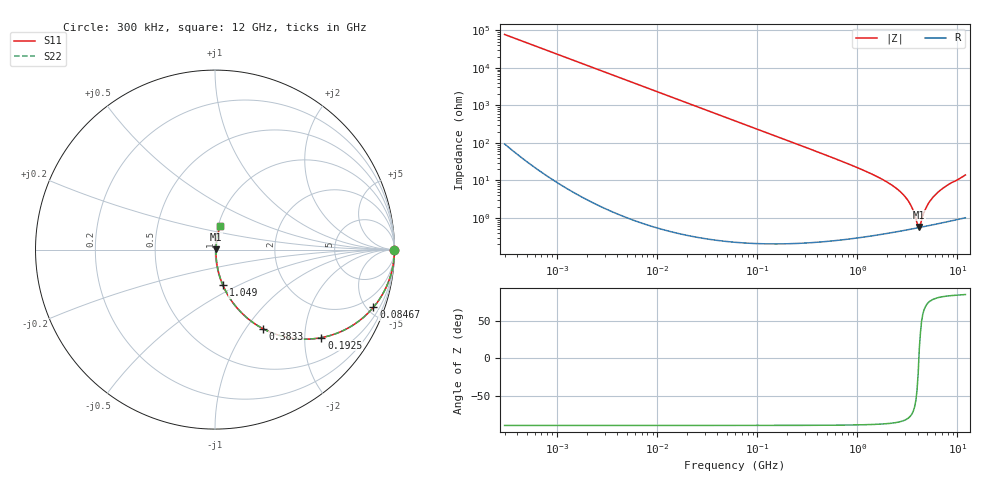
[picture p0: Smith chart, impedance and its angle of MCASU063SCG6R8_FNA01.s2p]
! MCASU063SCG6R8_FNA01  S-PARAMETER MODEL  ( Standard Model )
! Model Generated by TAIYO YUDEN Corporation (http://www.ty-top.com)
! Version 1.0
! TAIYO YUDEN Control No. 230609
! Copyright(c) 2023 TAIYO YUDEN CO.,LTD. All Rights Reserved.
! Product Description (link to TY-COMPAS)
! https://ds.yuden.co.jp/TYCOMPAS/or/detail?pn=MCASU063SCG6R8CFNA01&u=M
! Products Name : Multilayer Ceramic Capacitors
! Characteristics :
!  Capacitance : 6.8 [pF] , Rated Voltage : 50 [V] , TCC : CG / C0G
!  Case Size : 0.6 x 0.3 / 0.024 x 0.012 [mm/inch] , Thickness : 0.3 / 0.012 [mm/inch]
!  (Conditions: Temperature = 25 [degC] , DC Bias Voltage = 0 [V])
! External Node Assignments :
!  1  o---| |---o  2
! GND o---------o GND
! Frequency Range : 0.3MHz  -  12000MHz  [ 401 STEP ]
# MHZ S RI R 50
! Freq[MHz].  S11 Real  S11 Imag  S21 Real  S21 Imag  S12 Real  S12 Imag  S22 Real  S22 Imag
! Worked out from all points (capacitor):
!   401 points, 300 kHz to 12 GHz, reference 50 ohm
!   read as one part in series: C = 6.84 pF near 316.3 kHz
!   lowest |Z| = 571 mohm at 4.159 GHz (marker M1)
!   series resonance near 4.116 GHz, so ESL is about 220 pH
!   S11 on the Smith chart (normalised r, x): 300 kHz: open; 84.67 MHz: 1.00, -5.50; 192.5 MHz: 1.00, -2.41; 383.3 MHz: 1.00, -1.20; 1.049 GHz: 1.01, -0.42; 12 GHz: 1.02, +0.28
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0.3  1 -0.00129  3.21e-06 0.00129  3.21e-06 0.00129  1 -0.00129
1.769972  0.9999 -0.0076  5.99e-05 0.0076  5.99e-05 0.0076  0.9999 -0.0076
10.44266  0.998 -0.0448  0.00202 0.0448  0.00202 0.0448  0.998 -0.0448
27.10171  0.9866 -0.1148  0.0134 0.1148  0.0134 0.1148  0.9866 -0.1148
60  0.9376 -0.2416  0.0624 0.2416  0.0624 0.2416  0.9376 -0.2416
84.66778  0.8829 -0.3211  0.1171 0.3211  0.1171 0.3211  0.8829 -0.3211
192.4766  0.5929 -0.4905  0.4071 0.4905  0.4071 0.4905  0.5929 -0.4905
353.9943  0.2995 -0.4564  0.7005 0.4564  0.7005 0.4564  0.2995 -0.4564
383.2761  0.2669 -0.4405  0.7331 0.4405  0.7331 0.4405  0.2669 -0.4405
617.4538  0.1213 -0.3231  0.8787 0.3231  0.8787 0.3231  0.1213 -0.3231
1048.836  0.0439 -0.1979  0.9561 0.1979  0.9561 0.1979  0.0439 -0.1979
2088.533  0.0107 -0.0817  0.9893 0.0817  0.9893 0.0817  0.0107 -0.0817
2650.866  0.00701 -0.0509  0.993 0.0509  0.993 0.0509  0.00701 -0.0509
3107.553  0.00579 -0.032  0.9942 0.032  0.9942 0.032  0.00579 -0.032
3547.679  0.00537 -0.0169  0.9946 0.0169  0.9946 0.0169  0.00537 -0.0169
3944.255  0.00539 -0.00495  0.9946 0.00495  0.9946 0.00495  0.00539 -0.00495
4158.869  0.00552 0.00131  0.9945 -0.00131  0.9945 -0.00131  0.00552 0.00131
4270.516  0.00561 0.00388  0.9944 -0.00388  0.9944 -0.00388  0.00561 0.00388
5006.236  0.00652 0.0206  0.9935 -0.0206  0.9935 -0.0206  0.00652 0.0206
6026.253  0.0084 0.0406  0.9916 -0.0406  0.9916 -0.0406  0.0084 0.0406
8064.993  0.0136 0.0748  0.9864 -0.0748  0.9864 -0.0748  0.0136 0.0748
12000  0.0285 0.1342  0.9715 -0.1342  0.9715 -0.1342  0.0285 0.1342
